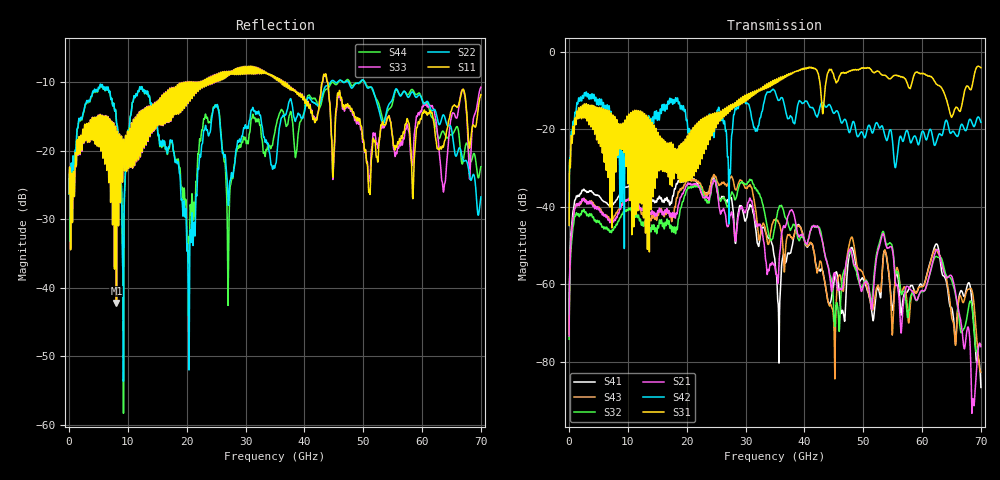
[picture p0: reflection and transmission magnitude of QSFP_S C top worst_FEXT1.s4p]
! AWR Design Environment (8415) Tue Jan 08 12:59:13 2019
! Document = 'QSFP Channel_S'
! nPorts: 4, nXvals: 7001
# HZ S DB R 50
!Freq DBS11 AngS11 DBS12 AngS12 DBS13 AngS13 DBS14 AngS14
!	DBS21 AngS21 DBS22 AngS22 DBS23 AngS23 DBS24 AngS24
!	DBS31 AngS31 DBS32 AngS32 DBS33 AngS33 DBS34 AngS34
!	DBS41 AngS41 DBS42 AngS42 DBS43 AngS43 DBS44 AngS44
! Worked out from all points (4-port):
!   7000 points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, 10 MHz to 70 GHz, reference 50 ohm
!   strongest paths, dB at 10 MHz, 17.51 GHz, 35.01 GHz, 52.51 GHz, 70 GHz:
!     S31: -44.8, -33.9, -7.3, -5.0, -4.0
!     S42: -44.8, -12.5, -10.2, -18.8, -18.2
!     S21: -73.4, -42.1, -55.5, -51.3, -76.1
!     S32: -74.2, -46.2, -45.1, -50.5, -75.6
!     S43: -72.8, -43.4, -43.4, -60.2, -82.7
!     S41: -69.9, -38.1, -54.2, -60.8, -86.7
!   lowest |S11| = -42.2 dB at 8.06 GHz (marker M1), VSWR 1.02, Z = 49.9 - j0.765 ohm
!   |S11| at or under -10 dB: start of sweep to 19.42 GHz; 36.78 GHz to 43.01 GHz (6.234 GHz wide, 15.6 % of centre); 43.97 GHz to end of sweep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
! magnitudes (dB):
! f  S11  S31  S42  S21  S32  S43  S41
! 10 MHz  -26.2  -44.8  -44.8  -73.4  -74.2  -72.8  -69.9
! 1.23 GHz  -22.1  -17.0  -14.4  -39.3  -41.5  -39.2  -37.2
! 8.06 GHz  -42.2  -18.4  -18.9  -42.7  -44.6  -41.5  -38.2
! 29.27 GHz  -7.7  -12.3  -12.2  -40.0  -33.7  -33.2  -39.7
! 45.02 GHz  -20.4  -6.2  -15.9  -57.2  -68.1  -70.9  -59.4
! 62.46 GHz  -19.0  -8.3  -23.0  -51.1  -52.8  -51.2  -49.6
! 70 GHz  -11.8  -4.0  -18.2  -76.1  -75.6  -82.7  -86.7
